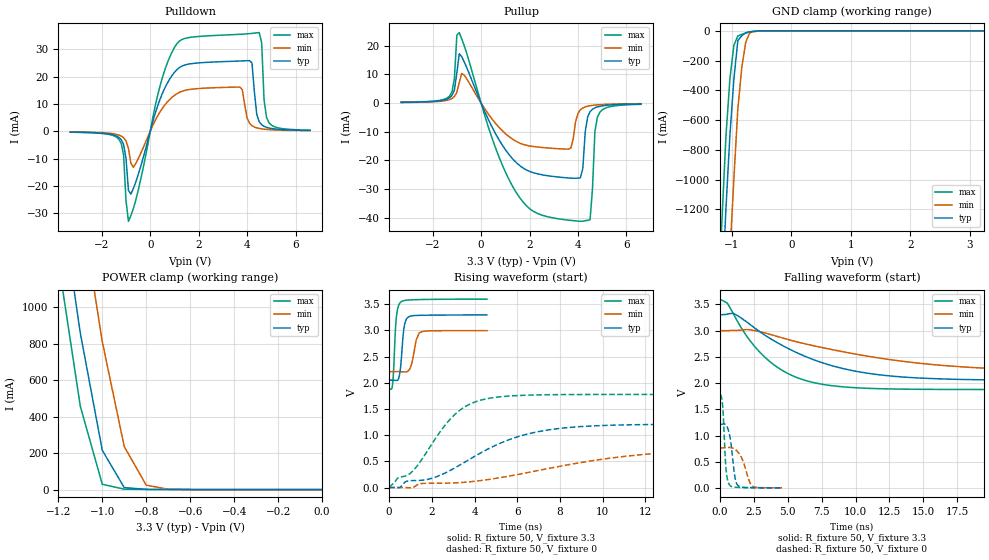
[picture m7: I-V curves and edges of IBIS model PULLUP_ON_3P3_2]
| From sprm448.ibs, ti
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|BUFFER OPERATING IN NORMAL MODE
|   Model Cell PULLUP_ON_3P3
|PULLUP_ON_3P3
[Model]   PULLUP_ON_3P3_2
Model_type   I/O
Polarity   Non-Inverting
Enable   Active-Low
Vinl =  0.8v
Vinh =  2v
Cref =  15.0000pF
Rref =  100.0000M
Vref =  0V
Vmeas =  1.65
C_comp   2.2653p   1.9017p   2.9162p
[Model Spec]
Vinl   0.8v   0.8v   0.8v
Vinh   2v   2v   2v
[Temperature Range]   25   125   -40
[Voltage Range]   3.3   3   3.6
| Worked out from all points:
|   slope of the pulldown table from 0 to 0.495 V, typ, clamps not added: 36.1 ohm
|   slope of the pullup table from 0 to 0.495 V, typ, clamps not added: 54.7 ohm
|   GND clamp passes 1 mA (typ) near -0.55 V on its own axis
|   POWER clamp passes 1 mA (typ) near -0.78 V on its own axis
|   rising waveform, R_fixture 50, V_fixture 3.3: 20-80 % time 160ps typ, 230ps min, 133ps max; typ from 2.05 V to 3.3 V
|   rising waveform, R_fixture 50, V_fixture 0: 20-80 % time 3.58ns typ, 6.73ns min, 1.95ns max; typ from 0.002 V to 1.21 V
|   falling waveform, R_fixture 50, V_fixture 3.3: 20-80 % time 6.15ns typ, 10.1ns min, 3.61ns max; typ from 3.3 V to 2.05 V
|   falling waveform, R_fixture 50, V_fixture 0: 20-80 % time 342ps typ, 611ps min, 212ps max; typ from 1.21 V to 0.004 V
[POWER_clamp]
|   voltage   I(typ)   I(min)   I(max)
-3.3V     22.02A     22.67A     21.68A
-1.2V     1.685A     2.433A     1.254A
-1.167V   1.409A     2.149A     988.2mA
-1.133V   1.134A     1.865A     722.7mA
-1.1V     858.4mA    1.581A     457.3mA
-1.033V   429.7mA    1.068A     171.9mA
-1V       215.3mA    810.7mA    29.21mA
-900mV    11.07mA    235.7mA    2.195mA
-800mV    1.113mA    24.41mA    1.221mA
-700mV    496.4uA    1.9mA      634.6uA
-11.55fV  39.74pA    5.746nA    488.5fA
[Pulldown]
|   voltage   I(typ)   I(min)   I(max)
-3.3V     -316.2uA   -252uA     -342.5uA
-1.3V     -2.195mA   -1.367mA   -2.881mA
-1.1V     -4.864mA   -2.357mA   -8.682mA
-900mV    -21.7mA    -6.326mA   -32.98mA
-700mV    -21.05mA   -13.22mA   -28.38mA
1.1V      22.53mA    13.73mA    32.03mA
3.7V      25.72mA    16.14mA    35.5mA
4.1V      25.85mA    2.912mA    35.75mA
4.5V      3.467mA    1.014mA    36.14mA
4.7V      1.789mA    754.6uA    11.41mA
4.9V      1.189mA    599.4uA    3.155mA
6.6V      300.9uA    215.3uA    389.5uA
[Pullup]
|   voltage   I(typ)   I(min)   I(max)
-3.3V     241.9uA    204.6uA    268.8uA
-1.3V     1.834mA    1.218mA    2.447mA
-1.1V     4.579mA    2.274mA    8.649mA
-900mV    17.22mA    7.132mA    24.6mA
500mV     -9.137mA   -6.074mA   -13.34mA
1.5V      -21.13mA   -13.59mA   -31.83mA
3.7V      -26.2mA    -15.78mA   -40.94mA
4.1V      -26.07mA   -2.353mA   -41.26mA
4.5V      -3.012mA   -927.6uA   -40.7mA
4.7V      -1.665mA   -705uA     -9.947mA
4.9V      -1.139mA   -567.3uA   -3.253mA
6.6V      -301.5uA   -210.8uA   -437.2uA
[GND_clamp]
|   voltage   I(typ)   I(min)   I(max)
-3.3V     -22.43A    -23.21A    -22A
-1.233V   -2.355A    -3.229A    -1.845A
-1.167V   -1.767A    -2.634A    -1.265A
-1.1V     -1.196A    -2.049A    -708.9mA
-1.033V   -702mA     -1.501A    -322.7mA
-966.7mV  -325.2mA   -993.1mA   -97.82mA
-900mV    -65.14mA   -524.7mA   -34.32mA
-833.3mV  -32.56mA   -245.5mA   -23.69mA
-766.7mV  -13.1mA    -75.12mA   -14.56mA
-700mV    -6.747mA   -13.52mA   -6.937mA
-433.3mV  -183.8uA   -314.6uA   -217.1uA
3.233V    -5.66uA    13.79uA    -45.87uA
[Ramp]
| variable   typ   min   max
dV/dt_f  0.7671239/6.178613n   0.4831527/10.20359n   1.058483/3.618502n
dV/dt_r  0.7313014/3.600882n   0.462791/6.841892n   1.071912/1.961425n
R_load = 50
[Rising Waveform]
R_fixture = 50
V_fixture = 3.3
V_fixture_min = 3
V_fixture_max = 3.6
|   time   V(typ)   V(min)   V(max)
0s        2.051V     2.214V     1.878V
152ps     2.051V     2.214V     1.948V
328ps     2.046V     2.214V     3.212V
456ps     2.098V     2.214V     3.49V
544ps     2.337V     2.213V     3.542V
688ps     3.032V     2.21V      3.57V
920ps     3.262V     2.239V     3.582V
1.272ns   3.287V     2.828V     3.588V
1.544ns   3.291V     2.98V      3.591V
4.576ns   3.297V     2.997V     3.599V
[Rising Waveform]
R_fixture = 50
V_fixture = 0
V_fixture_min = 0
V_fixture_max = 0
|   time   V(typ)   V(min)   V(max)
0s        2.058mV    1.646mV    2.756mV
392ps     -2.275mV   1.752mV    180.7mV
1.224ns   135mV      25.98mV    368.7mV
2.064ns   185.1mV    83.11mV    872.8mV
3.136ns   390.1mV    90.88mV    1.418V
4.704ns   752.3mV    157.8mV    1.706V
6.8ns     1.053V     311.9mV    1.768V
9.488ns   1.176V     511.6mV    1.778V
15.14ns   1.21V      714.7mV    1.779V
26.48ns   1.211V     762.3mV    1.779V
[Falling Waveform]
R_fixture = 50
V_fixture = 3.3
V_fixture_min = 3
V_fixture_max = 3.6
|   time   V(typ)   V(min)   V(max)
0s        3.3V       3V         3.6V
536ps     3.311V     3V         3.525V
1.056ns   3.319V     3.003V     3.288V
2.272ns   3.106V     3.015V     2.789V
3.832ns   2.83V      2.919V     2.377V
5.496ns   2.6V       2.798V     2.124V
7.672ns   2.377V     2.669V     1.972V
12.1ns    2.148V     2.464V     1.891V
19.14ns   2.063V     2.289V     1.878V
40.22ns   2.051V     2.217V     1.878V
[Falling Waveform]
R_fixture = 50
V_fixture = 0
V_fixture_min = 0
V_fixture_max = 0
|   time   V(typ)   V(min)   V(max)
0s        1.211V     765.4mV    1.779V
120ps     1.216V     765mV      1.719V
200ps     1.22V      765.6mV    1.556V
392ps     1.212V     769.4mV    563mV
472ps     1.19V      771mV      291.8mV
696ps     1.024V     773.4mV    62.87mV
1.128ns   171.2mV    734.5mV    15.41mV
1.336ns   46.72mV    681.1mV    12.16mV
2.432ns   7.608mV    29.66mV    5.169mV
4.6ns     3.813mV    4.654mV    3.447mV
